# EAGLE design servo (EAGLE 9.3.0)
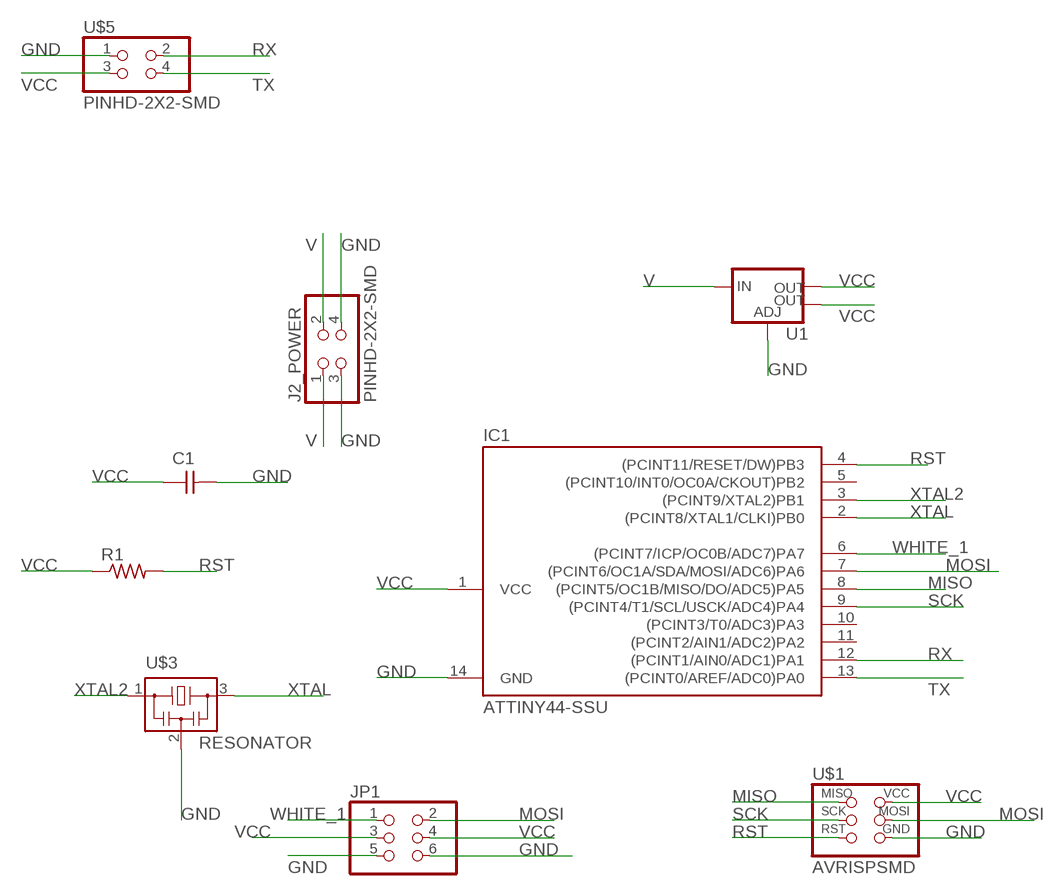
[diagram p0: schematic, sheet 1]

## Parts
C1  CAP-UNPOLARIZEDFAB  [C1206FAB]
IC1  ATTINY44-SSU  [SOIC14]
J2_POWER  PINHD-2X2-SMD  [2X02SMD]
JP1  PINHD-2X3-SMD  [2X03SMD]
R1  RES-US1206FAB  [R1206FAB]
U1  V_REG_LM1117SOT223  [SOT223]
U$1  AVRISPSMD  [2X03SMD]
U$3  RESONATOR  [EFOBM]
U$5  PINHD-2X2-SMD  [2X02SMD]

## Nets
GND: C1.2 IC1.14(GND) J2_POWER.3 J2_POWER.4 JP1.5 JP1.6 U1.1(ADJ) U$1.6(GND) U$3.2 U$5.1
MISO: IC1.8((PCINT5/OC1B/MISO/DO/ADC5)PA5) U$1.1(MISO)
MOSI: IC1.7((PCINT6/OC1A/SDA/MOSI/ADC6)PA6) JP1.2 U$1.4(MOSI)
RST: IC1.4((PCINT11/RESET/DW)PB3) R1.2 U$1.5(RST)
RX: IC1.12((PCINT1/AIN0/ADC1)PA1) U$5.2
SCK: IC1.9((PCINT4/T1/SCL/USCK/ADC4)PA4) U$1.3(SCK)
TX: IC1.13((PCINT0/AREF/ADC0)PA0) U$5.4
V: J2_POWER.1 J2_POWER.2 U1.3(IN)
VCC: C1.1 IC1.1(VCC) JP1.3 JP1.4 R1.1 U1.2(OUT) U1.4(OUT) U$1.2(VCC) U$5.3
WHITE_1: IC1.6((PCINT7/ICP/OC0B/ADC7)PA7) JP1.1
XTAL: IC1.2((PCINT8/XTAL1/CLKI)PB0) U$3.3
XTAL2: IC1.3((PCINT9/XTAL2)PB1) U$3.1
Unconnected: IC1.5((PCINT10/INT0/OC0A/CKOUT)PB2) IC1.10((PCINT3/T0/ADC3)PA3) IC1.11((PCINT2/AIN1/ADC2)PA2)

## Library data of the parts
C1 = eagle_fab:CAP-UNPOLARIZED
IC1 = eagle_fab:ATTINY44
J2_POWER U$5 = eagle_fab:PINHD-2X2-SMD
JP1 = eagle_fab:PINHD-2X3-SMD: PIN HEADER
R1 = eagle_fab:RES-US: Resistor (US Symbol)
U1 = eagle_fab:V_REG_LM1117: Voltage Regulator LM1117 Standard adjustable voltage regulator but in SMD form. Spark Fun Electronics SKU : COM-00595; PROD_ID: VREG-08170
U$1 = eagle_fab:AVRISP
U$3 = eagle_fab:RESONATOR

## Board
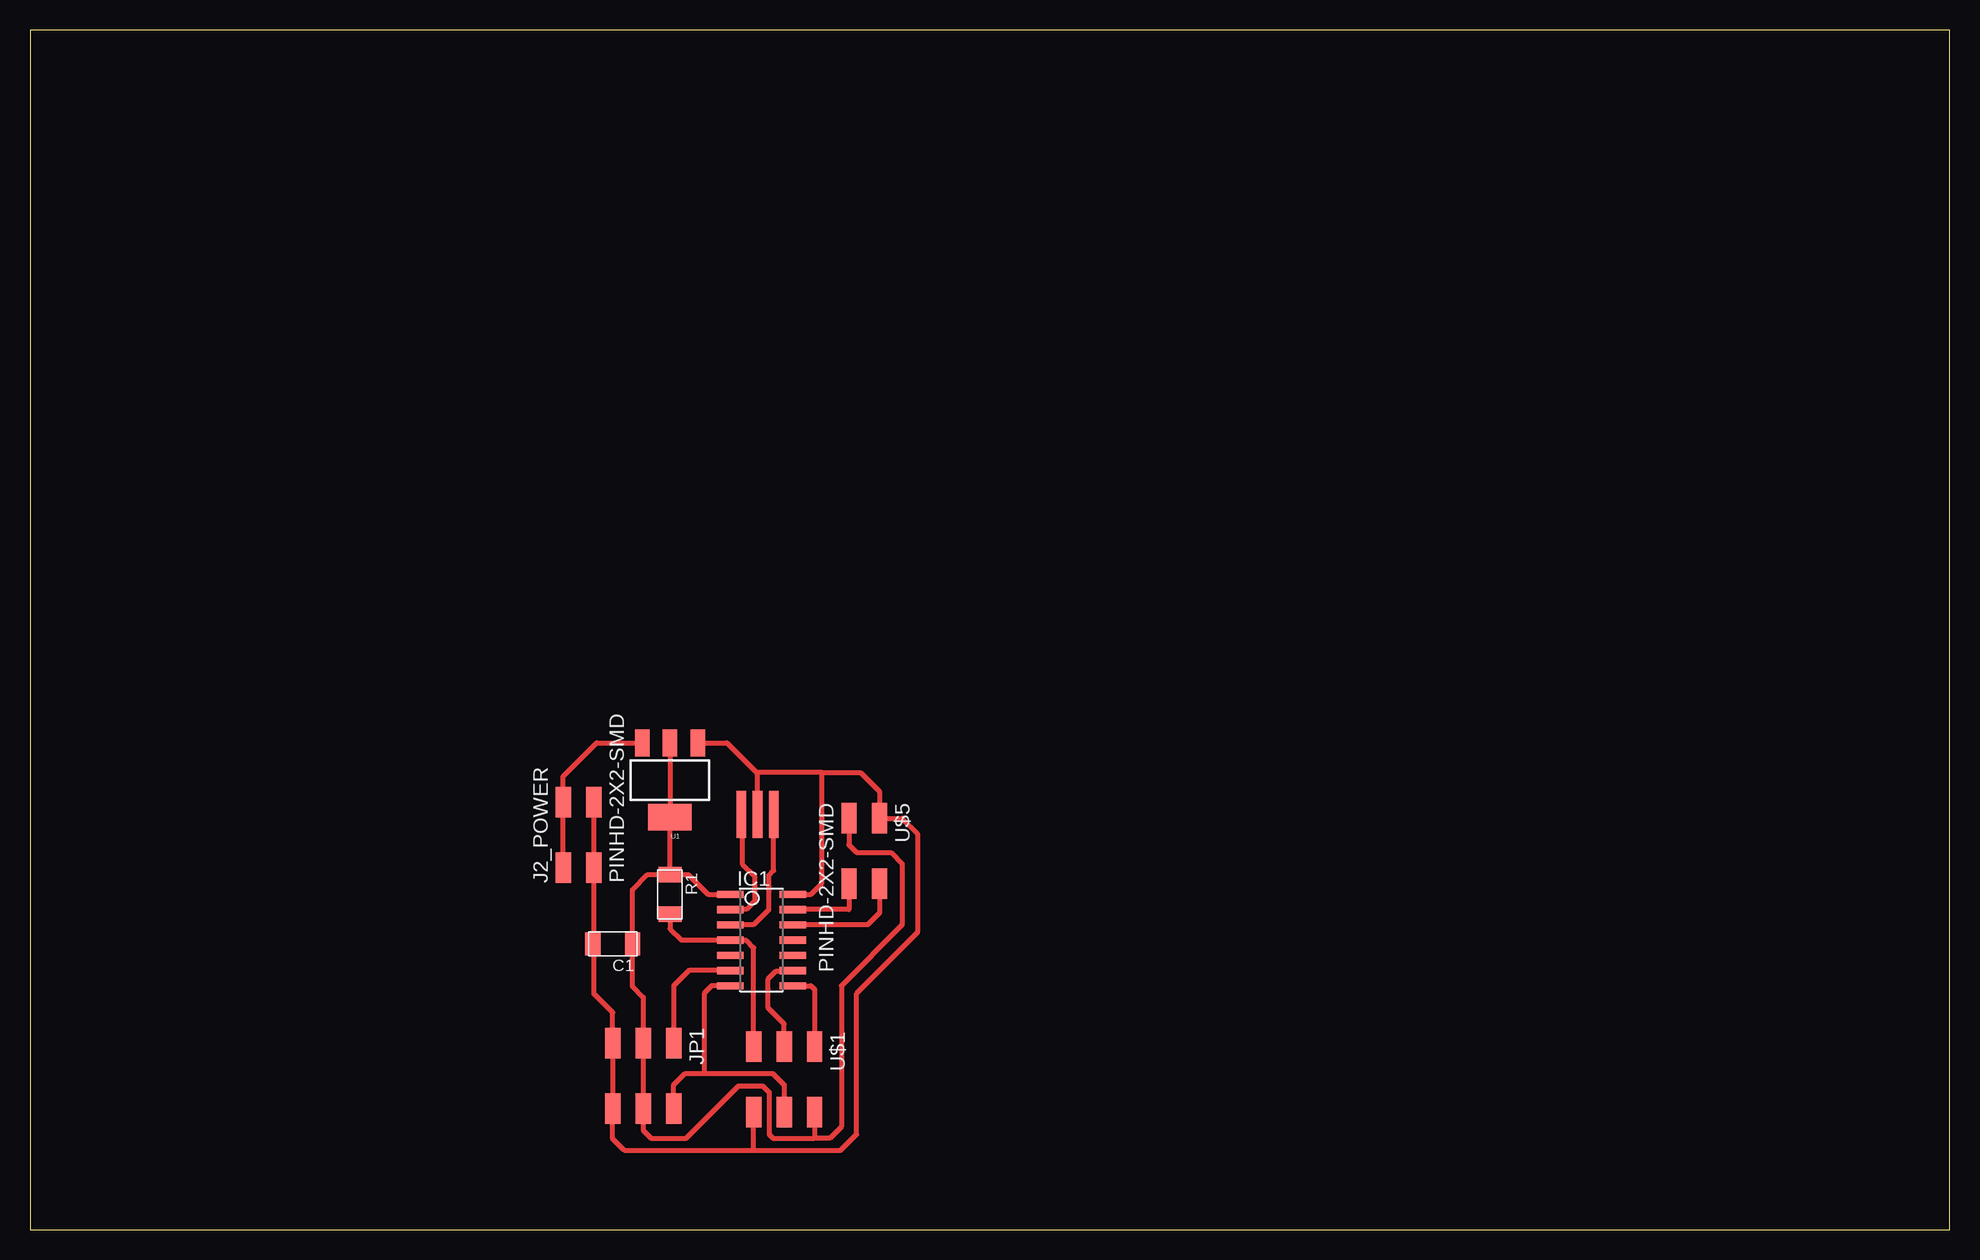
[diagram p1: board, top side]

Size 160 x 100 mm. Coordinates in mm from the lower left corner, seen from the top.
Outline: 0,0 160,0 160,100 0,100 0,0
Copper layers (1*16): Top 0.035mm / dielectric 1.5mm / Bottom 0.035mm
Design rules "eagle_fabcity-designrules *": minimum track width 16mil, minimum drill 32mil, track to track 16mil, track to pad 16mil, pad to pad 16mil, via to via 16mil, smd to smd 16mil, copper to edge 16mil, drill to drill 16mil, minimum pad ring 10mil, minimum via ring 8mil, stop-mask expansion 4mil, vias tented up to drill 0mil, thermal gap 16mil

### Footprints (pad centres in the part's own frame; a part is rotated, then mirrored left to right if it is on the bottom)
C1206FAB = smd 1.27 x 1.905: 1 -1.651,0; 2 1.651,0
SOIC14 = smd 0.61 x 2.21: 1 -3.81,-2.603; 2 -2.54,-2.603; 3 -1.27,-2.603; 4 0,-2.603; 5 1.27,-2.603; 6 2.54,-2.603; 7 3.81,-2.603; 8 3.81,2.603; 9 2.54,2.603; 10 1.27,2.603; 11 0,2.603; 12 -1.27,2.603; 13 -2.54,2.603; 14 -3.81,2.603
2X02SMD = smd 2.54 x 1.27: 1 -2.54,1.27; 2 2.92,1.27; 3 -2.54,-1.27; 4 2.92,-1.27
2X03SMD = smd 2.54 x 1.27: 1 -2.54,2.54; 2 2.92,2.54; 3 -2.54,0; 4 2.92,0; 5 -2.54,-2.54; 6 2.92,-2.54
R1206FAB = smd 1.27 x 1.905: 1 -1.651,0; 2 1.651,0
SOT223 = smd 1.219 x 2.235: 1 -2.311,-3.099; 2 0,-3.099; 3 2.311,-3.099 | smd 3.6 x 2.2: 4 0,3.099
EFOBM = smd 0.8 x 3.9: 1 -1.35,0; 2 0,0; 3 1.35,0

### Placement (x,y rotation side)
C1  48.58,23.81 180 top
IC1  60.96,24.13 270 top
J2_POWER  45.72,32.7 90 top
JP1  51.12,13.02 270 top
R1  53.34,27.94 270 top
U1  53.34,37.47 180 top
U$1  62.87,12.7 270 top
U$3  60.64,34.61 180 top
U$5  69.53,31.75 270 top

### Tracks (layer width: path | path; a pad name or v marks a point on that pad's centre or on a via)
GND
  Top 0.406: J2_POWER.4 J2_POWER.3 46.99,23.81 | 60.33,6.61 49.53,6.61 48.58,7.56 JP1.6 JP1.5 48.58,18.1 46.99,19.68 46.99,23.81 | U1.1 58.1,40.56 60.64,38.02 | 66.01,38.1 66.01,28.86 65.09,27.94 IC1.14 | U$3.2 60.64,38.02 | 46.99,23.81 C1.2 | 60.33,6.61 U$1.6 | 60.33,6.61 67.56,6.61 68.9,7.94 68.9,19.68 73.98,24.77 73.98,33.02 72.71,34.29 U$5.1 70.8,36.51 69.22,38.1 66.01,38.1 | 66.01,38.1 60.72,38.1 60.64,38.02
MISO
  Top 0.406: U$1.1 65.41,20 65.09,20.32 IC1.8
MOSI
  Top 0.406: 56.2,13.02 61.91,13.02 62.87,12.06 U$1.4 | IC1.7 56.83,20.32 56.2,19.68 56.2,13.02 | JP1.2 53.66,12.06 54.61,13.02 56.2,13.02
RST
  Top 0.406: U$1.5 60.33,23.48 59.71,24.09 58.4,24.09 IC1.4 54.29,24.13 53.34,25.08 R1.2
RX
  Top 0.406: U$5.2 70.8,26.38 69.82,25.4 IC1.12
SCK
  Top 0.406: U$1.3 62.87,17.14 61.53,18.48 61.53,20.88 62.21,21.55 63.52,21.55 IC1.9
TX
  Top 0.406: U$5.4 68.26,26.67 IC1.13
V
  Top 0.406: J2_POWER.1 J2_POWER.2 44.45,37.78 47.23,40.56 U1.3
VCC
  Top 0.406: U1.2 U1.4 R1.1 | IC1.1 56.52,27.94 54.86,29.59 R1.1 | U$1.2 65.41,7.62 | 65.41,7.62 66.67,7.62 67.63,8.57 67.63,20.32 72.71,25.4 72.71,30.48 71.75,31.43 68.9,31.43 68.26,32.07 U$5.3 | 65.41,7.62 61.91,7.62 61.91,7.63 61.61,7.94 61.61,11.44 61.08,11.98 59.05,11.98 54.7,7.62 51.75,7.62 51.12,8.26 JP1.4 JP1.3 51.12,19.37 50.23,20.26 C1.1 50.23,28.32 51.5,29.59 R1.1
WHITE_1
  Top 0.406: IC1.6 54.93,21.59 53.66,20.32 JP1.1
XTAL
  Top 0.406: IC1.2 58.4,26.71 59.71,26.71 60.39,27.38 60.39,29.46 59.37,30.48 59.37,34.53 U$3.3
XTAL2
  Top 0.406: IC1.3 58.4,25.44 60.35,25.44 61.59,26.68 61.59,29.53 61.99,29.93 U$3.1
